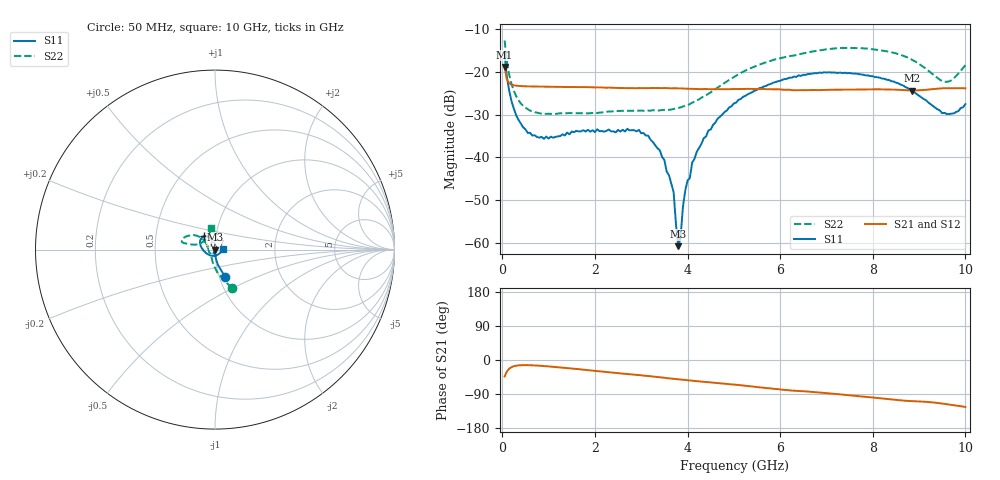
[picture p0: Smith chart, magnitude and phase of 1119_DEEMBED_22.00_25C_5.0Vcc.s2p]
!Hittite Microwave Corp.
!Digital Attenuator/PhaseShifter Rev 1.4.0
!Filename: C:\DATA\DATA\1119_DEEMBED_22.00_25C_5.0Vcc.s2p
!VNA ID: Agilent Technologies,N5224A,MY51441122,A.10.45.03
!Device type:
!2 Port Calibration.
!Temp(C): 25
!Lot Number:
!Serial Number:
!Operator:
!Misc:
!Attenuator:  22.000
# GHZ S DB R 50.0
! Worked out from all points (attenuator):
!   200 points, 50 MHz to 10 GHz, reference 50 ohm
!   highest |S21| = -18.82 dB at 50 MHz (marker M1); lowest = -24.3 dB at 8.85 GHz (marker M2)
!   lowest |S11| = -60.8 dB at 3.8 GHz (marker M3), VSWR 1.00, Z = 50 - j0.09 ohm
!   |S11| at or under -10 dB: start of sweep to end of sweep
!   |S22| runs from -29.8 to -12.6 dB; largest |S21 - S12| = 0.00017
!   S11 on the Smith chart (normalised r, x): 50 MHz: 1.06, -0.33; 6.7 GHz: 0.88, +0.13; 10 GHz: 1.09, +0.00
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0.05  -15.84 -69.8  -18.82 -43.3  -18.82 -43.4  -12.60 -66.5
0.1  -21.23 -79.1  -21.78 -30.3  -21.77 -30.3  -17.56 -83.4
0.2  -26.84 -84.8  -22.95 -18.8  -22.95 -18.8  -22.84 -100.2
0.55  -34.28 -91.3  -23.37 -13.6  -23.36 -13.6  -28.72 -125.8
1  -35.61 -98.9  -23.45 -16.9  -23.46 -16.9  -29.78 -136.3
1.75  -33.64 -109.3  -23.54 -25.5  -23.54 -25.5  -29.66 -139.7
2.95  -33.58 -100.9  -23.76 -39.7  -23.77 -39.8  -29.07 -158.7
3.4  -38.32 -103.9  -23.77 -45.5  -23.78 -45.5  -29.00 -172.1
3.7  -48.20 -97.9  -23.81 -49.6  -23.82 -49.6  -28.67 176.7
3.8  -60.84 -82.4  -23.84 -51.0  -23.85 -51.0  -28.45 172.1
3.85  -58.69 112.6  -23.86 -51.6  -23.86 -51.6  -28.30 170.0
3.9  -51.69 79.9  -23.86 -52.3  -23.87 -52.3  -28.10 168.2
3.95  -47.83 81.0  -23.90 -53.0  -23.91 -53.0  -27.88 165.7
4.05  -44.84 80.0  -23.93 -53.9  -23.94 -54.0  -27.51 161.4
4.1  -41.25 86.9  -23.92 -54.6  -23.92 -54.7  -27.20 159.7
4.45  -33.69 86.0  -24.03 -58.8  -24.05 -58.8  -25.09 147.5
5.05  -27.17 99.2  -23.99 -65.3  -24.01 -65.3  -20.85 139.5
6.7  -20.36 129.5  -24.22 -84.4  -24.24 -84.5  -15.19 154.5
8.35  -21.87 167.3  -24.11 -103.6  -24.11 -103.6  -15.24 168.1
8.85  -24.49 -170.3  -24.34 -108.5  -24.34 -108.5  -17.14 167.8
9.55  -29.58 -81.6  -23.80 -116.0  -23.82 -116.0  -22.28 138.8
10  -27.53 2.1  -23.83 -123.8  -23.83 -123.8  -18.39 99.5
